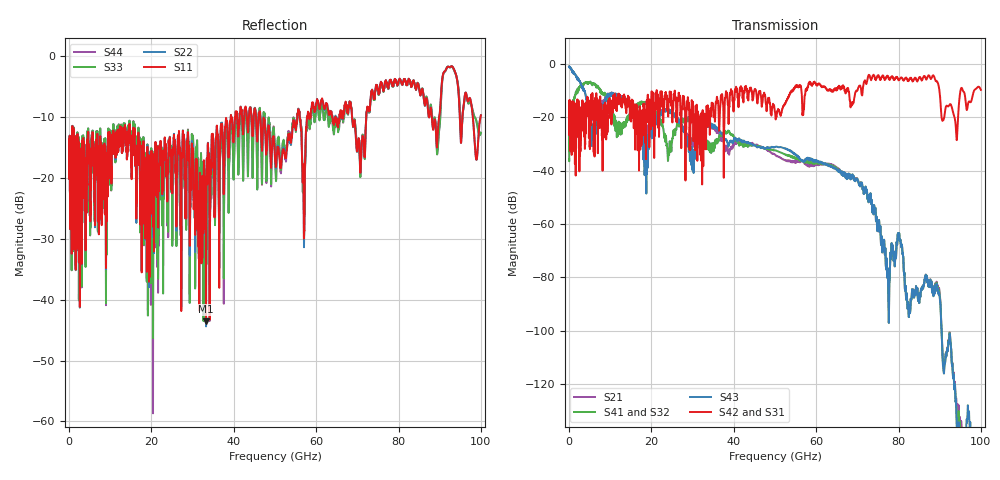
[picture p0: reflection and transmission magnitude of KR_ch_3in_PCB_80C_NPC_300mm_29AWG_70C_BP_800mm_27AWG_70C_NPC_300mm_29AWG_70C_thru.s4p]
# GHz S RI R 45
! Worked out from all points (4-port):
!   4000 points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, 25 MHz to 100 GHz, reference 45 ohm
!   strongest paths, dB at 25 MHz, 25.02 GHz, 50.02 GHz, 75.03 GHz, 100 GHz:
!     S42: -20.0, -17.9, -18.0, -4.4, -9.7
!     S31: -20.0, -18.0, -18.1, -4.4, -9.7
!     S43: -0.9, -17.9, -31.2, -59.9, -157.0
!     S41: -35.7, -29.0, -32.4, -59.9, -162.9
!     S32: -35.7, -29.1, -32.4, -59.9, -162.8
!     S21: -0.9, -17.7, -34.0, -60.0, -173.5
!   lowest |S11| = -43.6 dB at 33.27 GHz (marker M1), VSWR 1.01, Z = 44.9 + j0.579 ohm
!   |S11| at or under -10 dB: start of sweep to 39.26 GHz; 46.41 GHz to 55.4 GHz (8.984 GHz wide, 17.6 % of centre); 68.72 GHz to 72.15 GHz (3.432 GHz wide, 4.87 % of centre)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
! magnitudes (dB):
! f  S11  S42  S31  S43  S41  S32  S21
! 25 MHz  -16.0  -20.0  -20.0  -0.9  -35.7  -35.7  -0.9
! 4.725 GHz  -14.5  -13.5  -13.5  -15.1  -7.4  -7.4  -14.2
! 18.68 GHz  -24.1  -35.7  -35.7  -33.1  -14.5  -14.5  -26.0
! 33.27 GHz  -43.6  -27.7  -28.3  -22.5  -29.4  -29.4  -22.3
! 69.55 GHz  -12.1  -10.6  -10.6  -44.0  -43.8  -43.8  -43.7
! 77.42 GHz  -4.8  -4.8  -4.8  -79.4  -79.5  -79.5  -79.5
! 100 GHz  -9.7  -9.7  -9.7  -157.0  -162.9  -162.8  -173.5
